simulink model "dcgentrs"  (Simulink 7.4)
settings: Solver=ode45  StartTime=0.0  StopTime=10  MaxStep=0.05  RelTol=1e-3

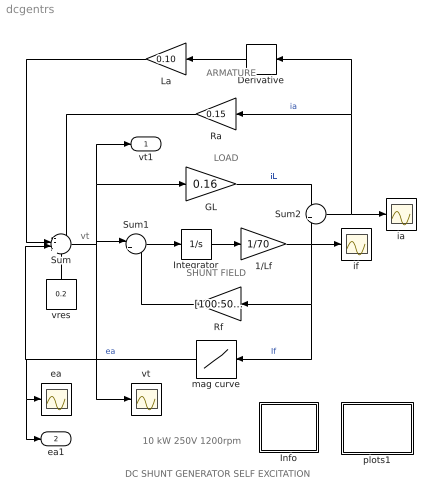
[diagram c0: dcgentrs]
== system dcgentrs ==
  note: vt
  note: DC SHUNT GENERATOR SELF EXCITATION
  note: 10 kW 250V 1200rpm
  note: ARMATURE
  note: SHUNT FIELD
  note: LOAD
  1/Lf : Gain  Gain=1/70  ParameterDataType=sfix(16)  ParameterScaling=2^0  OutDataType=sfix(16)  OutScaling=2^0
  Derivative : Derivative
  GL : Gain  Gain=0.16  ParameterDataType=sfix(16)  ParameterScaling=2^0  OutDataType=sfix(16)  OutScaling=2^0
  Info : Subsystem
  Integrator : Integrator
  La : Gain  Gain=0.10  ParameterDataType=sfix(16)  ParameterScaling=2^0  OutDataType=sfix(16)  OutScaling=2^0
  Ra : Gain  Gain=0.15  ParameterDataType=sfix(16)  ParameterScaling=2^0  OutDataType=sfix(16)  OutScaling=2^0
  Rf : Gain  Gain=[100:50:300]  ParameterDataType=sfix(16)  ParameterScaling=2^0  OutDataType=sfix(16)  OutScaling=2^0
  Sum : Sum  Inputs=--++  OutDataType=sfix(16)  OutScaling=2^0
  Sum1 : Sum  Inputs=|+-  OutDataType=sfix(16)  OutScaling=2^0
  Sum2 : Sum  OutDataType=sfix(16)  OutScaling=2^0
  ea : Scope
  ia : Scope
  if : Scope
  mag curve : Lookup  InputValues=[0 .4 .5 .6 .7 .8 1 1.2 1.4 1.6 1.8 2 2.2 2.4 2.8 3.0]  Table=[0 140 162 176 189 200 216 226 237 247 256 260 265 270 275 276]  OutDataType=sfix(16)  OutScaling=2^0
  plots1 : Subsystem
  vres : Constant  Value=0.2  OutDataType=sfix(16)  OutScaling=2^0
  vt : Scope
  vt1 : Outport
  ea1 : Outport  Port=2
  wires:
  Sum1/1 -> Integrator/1
  Sum/1 -> Sum1/1, vt/1, GL/1, vt1/1
  GL/1 -> Sum2/1  "iL"
  Integrator/1 -> 1/Lf/1
  1/Lf/1 -> Sum2/2, if/1, mag curve/1, Rf/1  "If"
  Rf/1 -> Sum1/2
  vres/1 -> Sum/4
  mag curve/1 -> Sum/3, ea/1, ea1/1  "ea"
  Derivative/1 -> La/1
  La/1 -> Sum/2
  Ra/1 -> Sum/1
  Sum2/1 -> Derivative/1, Ra/1, ia/1  "ia"

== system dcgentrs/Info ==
  note: This demonstration illustrates the current and voltage buildup in a self-excited dc shunt generator driven at constant speed. Examine the effects of: a) changing the residual voltage magnitude and polarity (vres) b) varying the field resistance Rf =[145 200 250 300 350] c) varying the load conductance GL=[0.16 0.5 ] d) changing the field inductance Lf e) modifying the armature parameters Ra and La
  note: Self-excited dc generator
  note: System equations: ea = vt + Ra ia + La dia/dt = g(if) (armature) vt = Rf if + Lf dif/dt (field) iL = GL vt ia= iL + if (load)
  note: Nomenclature: Ra = armature resistance [ohms] La = armature inductance [H] Rf = fileld resistance [ohms] Lf = field inductance [H] GL = load conductance [mhos] vt = terminal voltage [V] ea = open-circuit voltage [V] vres = residual voltage [v] if = field current [A] iL = load current [A] ia = armature current [A]

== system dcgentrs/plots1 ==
